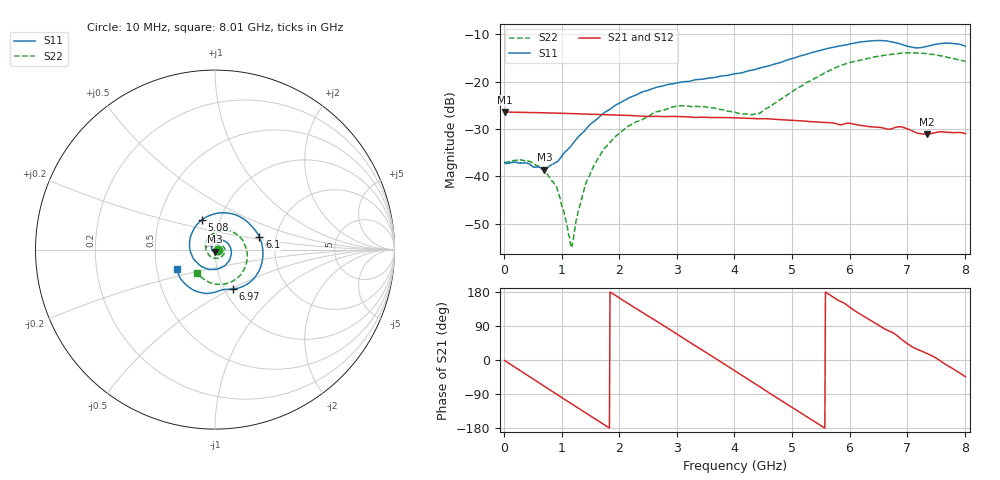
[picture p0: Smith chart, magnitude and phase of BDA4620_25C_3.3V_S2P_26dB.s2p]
!Agilent Technologies,E5071B,MY42404982,A.09.10
!Date: Wed May 06 08:54:28 2026
!Data & Calibration Information:
!Freq	S11:SOLT2(ON)	S21:SOLT2(ON)	S12:SOLT2(ON)	S22:SOLT2(ON)
# Hz S RI R 50
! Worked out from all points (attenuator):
!   801 points, 10 MHz to 8.01 GHz, reference 50 ohm
!   highest |S21| = -26.37 dB at 10 MHz (marker M1); lowest = -31.1 dB at 7.34 GHz (marker M2)
!   lowest |S11| = -38.6 dB at 700 MHz (marker M3), VSWR 1.02, Z = 49.7 - j1.14 ohm
!   |S11| at or under -10 dB: start of sweep to end of sweep
!   |S22| runs from -54.7 to -13.9 dB; largest |S21 - S12| = 0.00022
!   S11 on the Smith chart (normalised r, x): 10 MHz: 1.03, -0.00; 5.08 GHz: 0.82, +0.28; 6.1 GHz: 1.64, +0.24; 6.97 GHz: 1.09, -0.51; 8.01 GHz: 0.64, -0.14
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1e7  0.0141 -0.000909  0.048 -0.001  0.0481 -0.000988  0.014 -0.000452
4.2e8  0.00845 -0.0108  0.0352 -0.0315  0.0353 -0.0316  0.0136 -0.00494
7e8  -0.00267 -0.0114  0.0165 -0.0439  0.0165 -0.0439  0.00897 -0.00708
9.3e8  -0.0132 -0.00577  -0.00159 -0.0465  -0.00161 -0.0465  0.0035 -0.00628
1.16e9  -0.0197 0.00678  -0.0191 -0.0419  -0.0192 -0.042  -0.00147 -0.00114
1.2e9  -0.0203 0.00946  -0.0219 -0.0405  -0.0219 -0.0405  -0.00208 -1.95e-05
1.35e9  -0.0202 0.02  -0.0312 -0.0334  -0.0312 -0.0335  -0.00359 0.0046
1.53e9  -0.015 0.0336  -0.0394 -0.0224  -0.0395 -0.0224  -0.0035 0.0112
1.77e9  0.000898 0.0482  -0.0446 -0.00491  -0.0447 -0.00493  0.000627 0.0205
2.15e9  0.0405 0.0527  -0.038 0.0224  -0.038 0.0225  0.0169 0.0292
2.68e9  0.088 0.00649  -0.00689 0.0424  -0.00686 0.0425  0.0442 0.0196
3.08e9  0.0822 -0.0556  0.0209 0.0372  0.021 0.0373  0.0552 -0.00725
4.01e9  -0.0795 -0.0913  0.0363 -0.0201  0.0364 -0.0201  -0.0103 -0.0465
4.43e9  -0.1387 -0.00418  0.0143 -0.038  0.0142 -0.0381  -0.0447 -0.0117
5.08e9  -0.071 0.1673  -0.0264 -0.0285  -0.0265 -0.0285  -0.0213 0.082
5.35e9  0.0138 0.2032  -0.0352 -0.0137  -0.0353 -0.0137  0.0228 0.1019
6.1e9  0.2475 0.0687  -0.0222 0.0275  -0.0222 0.0275  0.1594 0.042
6.68e9  0.2015 -0.1759  0.00712 0.0307  0.00718 0.0307  0.1703 -0.0899
6.97e9  0.0982 -0.2198  0.0222 0.0235  0.0223 0.0235  0.1307 -0.1532
7.34e9  0.00756 -0.2351  0.0266 0.00831  0.0267 0.0084  0.0429 -0.1931
7.66e9  -0.1154 -0.2279  0.0288 -0.00558  0.0289 -0.00553  -0.0353 -0.1804
8.01e9  -0.212 -0.1066  0.0203 -0.0197  0.0204 -0.0197  -0.1018 -0.1276
